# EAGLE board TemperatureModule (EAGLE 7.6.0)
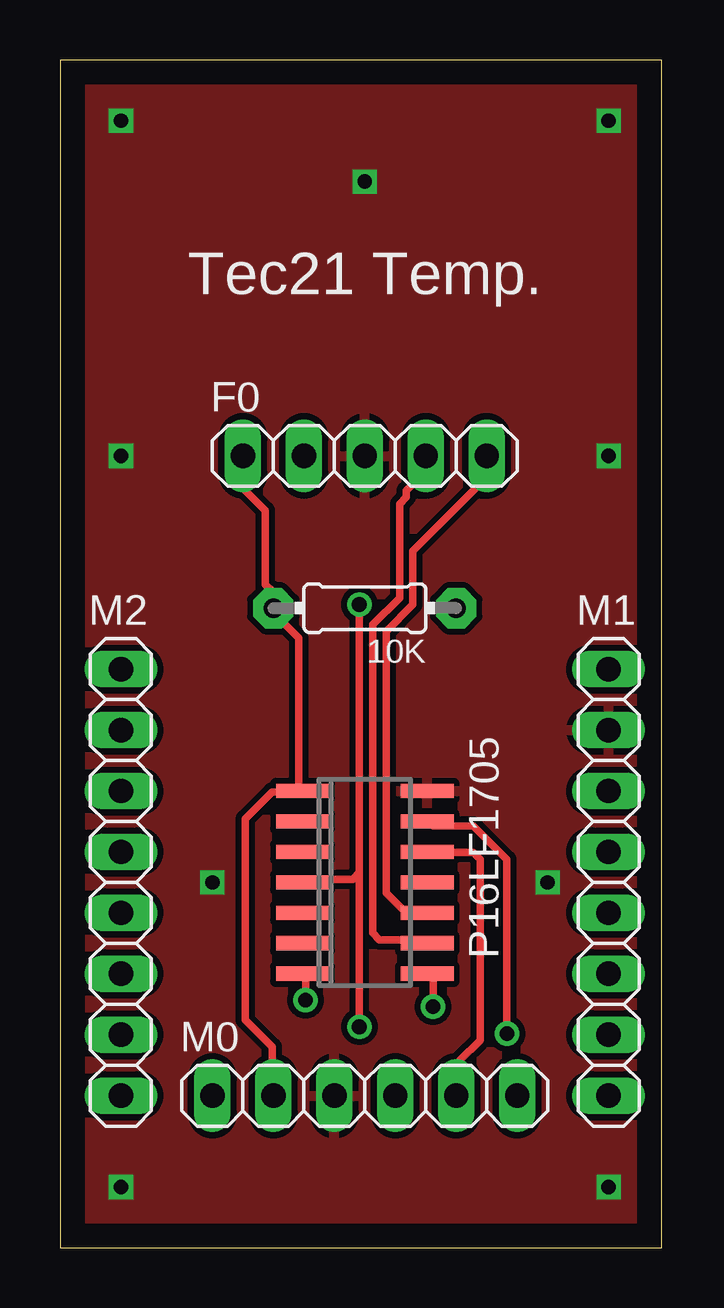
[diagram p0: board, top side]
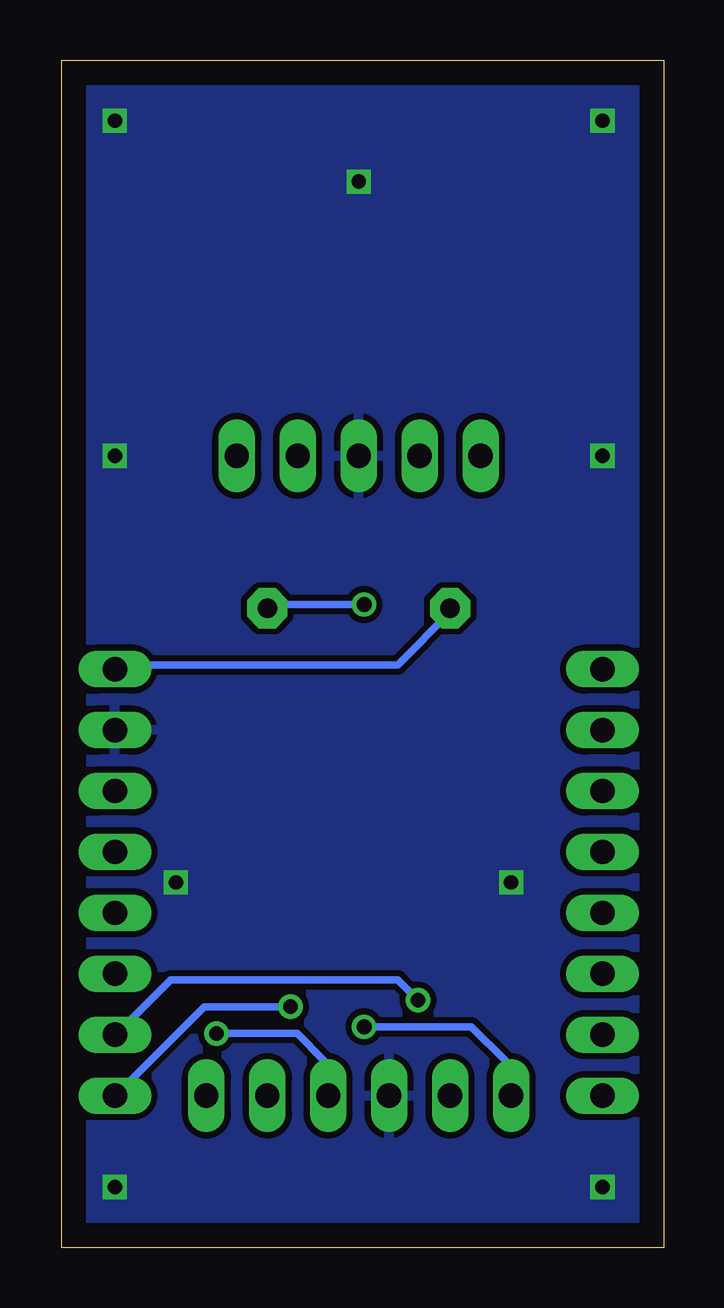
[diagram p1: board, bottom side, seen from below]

Size 25.07 x 49.52 mm. Coordinates in mm from the lower left corner, seen from the top.
Outline: 0,0 25.07,0 25.07,49.52 0,49.52 0,0
Copper layers (1*16): Top 0.035mm / dielectric 1.5mm / Bottom 0.035mm
Design rules "default": minimum track width 10mil, minimum drill 24mil, track to track 8mil, track to pad 8mil, pad to pad 8mil, via to via 8mil, smd to smd 8mil, copper to edge 40mil, drill to drill 8mil, minimum pad ring 10mil, minimum via ring 8mil, stop-mask expansion 4mil, vias tented up to drill 0mil, thermal gap 10mil
Net classes: 0 default: width 0.305 mm, drill 0.61 mm, clearance 0.254 mm

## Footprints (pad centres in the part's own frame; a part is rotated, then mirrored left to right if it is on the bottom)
0204/7 = drill 0.813 pad 1.676 octagon: 1 -3.81,0; 2 3.81,0
1X05 = drill 1.016 long: 1 -5.08,0; 2 -2.54,0; 3 0,0; 4 2.54,0; 5 5.08,0
1X06 = drill 1.016 long: 1 -6.35,0; 2 -3.81,0; 3 -1.27,0; 4 1.27,0; 5 3.81,0; 6 6.35,0
1X08 = drill 1.016 long: 1 -8.89,0; 2 -6.35,0; 3 -3.81,0; 4 -1.27,0; 5 1.27,0; 6 3.81,0; 7 6.35,0; 8 8.89,0
SO-14 = smd 0.6 x 2.2: 1 -3.81,-2.6; 2 -2.54,-2.6; 3 -1.27,-2.6; 4 0,-2.6; 5 1.27,-2.6; 6 2.54,-2.6; 7 3.81,-2.6; 8 3.81,2.6; 9 2.54,2.6; 10 1.27,2.6; 11 0,2.6; 12 -1.27,2.6; 13 -2.54,2.6; 14 -3.81,2.6

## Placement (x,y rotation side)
10K  10k  [0204/7]  12.7,26.67 180 top
F0  [1X05]  12.7,33.02 0 top
M0  [1X06]  12.7,6.35 0 top
M1  [1X08]  22.86,15.24 270 top
M2  [1X08]  2.54,15.24 270 top
P16LF1705  PIC16F676SL  [SO-14]  12.7,15.24 270 top

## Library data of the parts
10K = adafruit
F0 M0 M1 M2 = pinhead
P16LF1705 = microchip; MF: MICROCHIP; MPN: PIC16F676-I/SL; OC_FARNELL: 9760520; OC_NEWARK: 92C4557

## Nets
CCL: M1.7 P16LF1705.7
CDA: M1.8 P16LF1705.8
GND: F0.3 M0.3 M1.2 P16LF1705.14
LCL: F0.5 P16LF1705.10
LDA: F0.4 P16LF1705.9
MCLR: 10K.1 M0.1 P16LF1705.4
O3: F0.2
PGC: M0.5 P16LF1705.12
PGD: M0.4 P16LF1705.13
VDD: 10K.2 F0.1 M0.2 M1.1 P16LF1705.1

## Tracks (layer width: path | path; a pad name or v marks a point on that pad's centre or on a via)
CCL  (via drill 0.61)
  Top 0.305: v10.24,10.34 10.24,11.18 P16LF1705.7
  Bottom 0.305: v10.24,10.34 11.07,11.18 20.52,11.18 22.76,8.94 22.61,8.94 M1.7
CDA  (via drill 0.61)
  Top 0.305: v15.54,10.06 15.54,11.18 P16LF1705.8
  Bottom 0.305: v15.54,10.06 19.13,10.06 22.76,6.43 22.61,6.43 M1.8
GND  (via drill 0.6)
  other vias: 2.54,46.99 2.54,33.02 2.54,2.54 22.86,2.54 22.86,33.02 22.86,46.99 12.7,44.45 6.35,15.24 20.32,15.24
  pour Top: -1.27,50.8 26.67,50.8 26.67,-1.27 -1.27,-1.27
  pour Bottom: -1.27,50.8 26.67,50.8 26.67,-1.27 -1.27,-1.27
LCL
  Top 0.305: P16LF1705.10 14.43,13.97 13.59,14.81 13.59,25.7 14.71,26.82 14.71,29.06 17.78,32.13 F0.5
LDA
  Top 0.305: P16LF1705.9 15.27,12.85 13.31,12.85 13.03,13.13 13.03,25.98 14.15,27.1 14.15,31.01 14.43,31.29 14.43,31.57 14.99,32.13 14.99,32.97 F0.4
MCLR  (via drill 0.61)
  Top 0.305: 12.47,15.65 12.19,15.37 10.24,15.37 P16LF1705.4 | v12.47,26.82 12.47,15.65 | 12.47,15.65 v12.47,9.22
  Bottom 0.305: v12.47,26.82 16.38,26.82 10K.1 | v12.47,9.22 8,9.22 6.6,7.82 6.6,6.43 M0.1
PGC
  Top 0.305: P16LF1705.12 15.54,16.48 17.22,16.48 17.5,16.2 17.5,8.66 16.66,7.82 16.66,6.43 M0.5
PGD  (via drill 0.61)
  Top 0.305: v18.62,8.94 18.62,16.2 17.22,17.6 15.54,17.6 P16LF1705.13
  Bottom 0.305: v18.62,8.94 15.27,8.94 14.15,7.82 14.15,6.43 M0.4
VDD
  Top 0.305: F0.1 7.72,32.97 7.72,31.57 8.56,30.73 8.56,27.66 8.84,27.38 8.84,26.82 10K.2 9.12,26.54 9.12,26.26 9.96,25.43 9.96,19.28 P16LF1705.1 9.96,19 8.84,19 7.72,17.88 7.72,9.5 8.84,8.38 8.84,6.43 M0.2
  Bottom 0.305: M1.1 21.34,24.31 11.07,24.31 8.84,26.54 10K.2

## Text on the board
tPlace: Tec21 Temp.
